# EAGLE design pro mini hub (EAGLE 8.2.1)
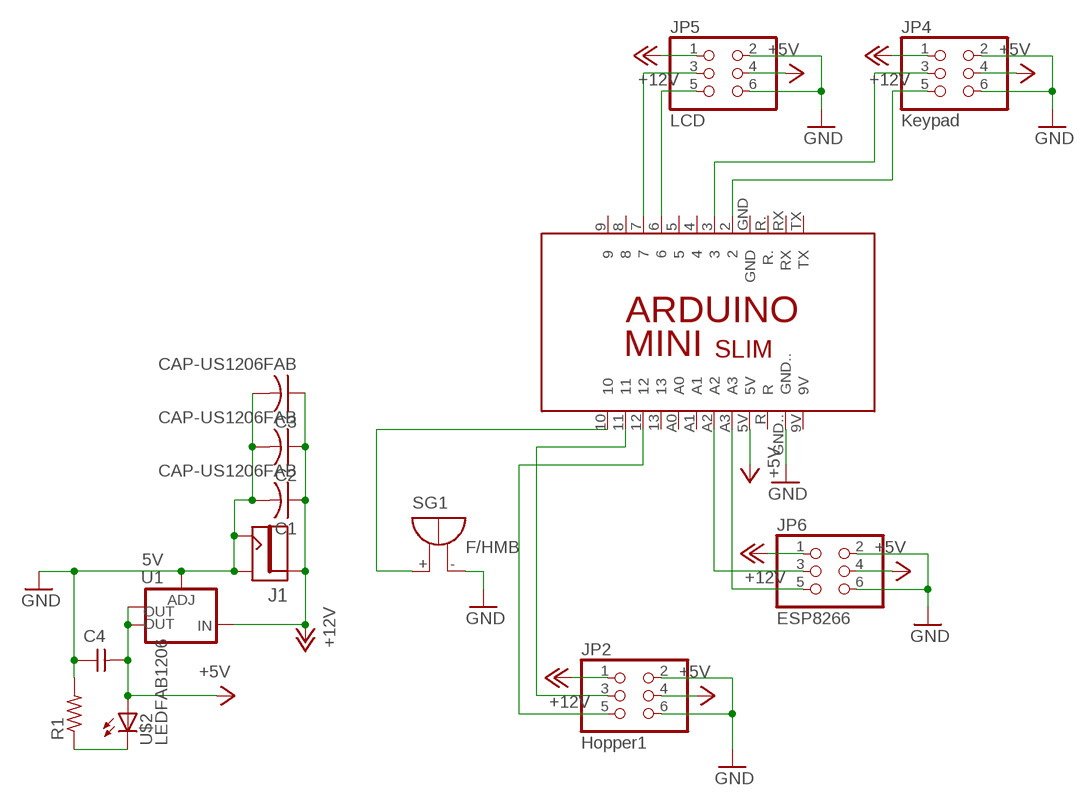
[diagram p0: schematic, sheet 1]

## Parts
C1  CAP-US1206FAB  [C1206FAB]
C2  CAP-US1206FAB  [C1206FAB]
C3  CAP-US1206FAB  [C1206FAB]
C4  CAP-UNPOLARIZEDFAB  [C1206FAB]
J1  JACK2.1MM  [JACK_2.1MM]
JP2  Hopper1  PINHD-2X3-SMD  [2X03SMD]
JP4  Keypad  PINHD-2X3-SMD  [2X03SMD]
JP5  LCD  PINHD-2X3-SMD  [2X03SMD]
JP6  ESP8266  PINHD-2X3-SMD  [2X03SMD]
PCB1  ARDUINO_MINI_SLIM  [ARDUINO_MINI_SLIM]
R1  RES-US1206FAB  [R1206FAB]
SG1  F/HMB  [F/HMB]
U1  5V  V_REG_LM1117SOT223  [SOT223]
U$2  LEDFAB1206  [LED1206FAB]

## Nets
+5V: C4.2 JP2.4 JP4.4 JP5.4 JP6.4 PCB1.5V U1.2(OUT) U1.4(OUT) U$2.1(A)
+12V: C1.1 C2.1 C3.1 J1.PIN JP2.1 JP4.1 JP5.1 JP6.1 U1.3(IN)
GND: C1.2 C2.2 C3.2 C4.1 J1.CONTACT J1.SHUNT JP2.2 JP2.6 JP4.2 JP4.6 JP5.2 JP5.6 JP6.2 JP6.6 PCB1.GND.. R1.2 SG1.- U1.1(ADJ)
N$1: PCB1.10 SG1.+
N$2: R1.1 U$2.2(C)
N$3: JP2.3 PCB1.11
N$4: JP2.5 PCB1.12
N$5: JP6.5 PCB1.A3
N$6: JP6.3 PCB1.A2
N$7: JP5.5 PCB1.6
N$8: JP5.3 PCB1.7
N$9: JP4.5 PCB1.2
N$10: JP4.3 PCB1.3
Unconnected: PCB1.4 PCB1.5 PCB1.8 PCB1.9 PCB1.9V PCB1.13 PCB1.A0 PCB1.A1 PCB1.GND PCB1.R PCB1.R. PCB1.RX PCB1.TX

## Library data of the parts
C1-C3 = fab:CAP-US
C4 = fab:CAP-UNPOLARIZED
J1 = fab:JACK
JP2 JP4-JP6 = fab:PINHD-2X3-SMD: PIN HEADER
PCB1 = E14_Arduino_revC:ARDUINO_MINI_SLIM: Device for representing an Arduino Mini board with a footprint in an EAGLE design. Created by Dave Young for Element14. More EAGLE documentation at: http://www.element14.com/community/community/knode/cadsoft_eagle
R1 = fab:RES-US: Resistor (US Symbol)
SG1 = buzzer:F/HMB: BUZZER; OC_FARNELL: unknown; OC_NEWARK: unknown
U1 = fab:V_REG_LM1117: Voltage Regulator LM1117 Standard adjustable voltage regulator but in SMD form. Spark Fun Electronics SKU : COM-00595; PROD_ID: VREG-08170
U$2 = fab:LED: LED

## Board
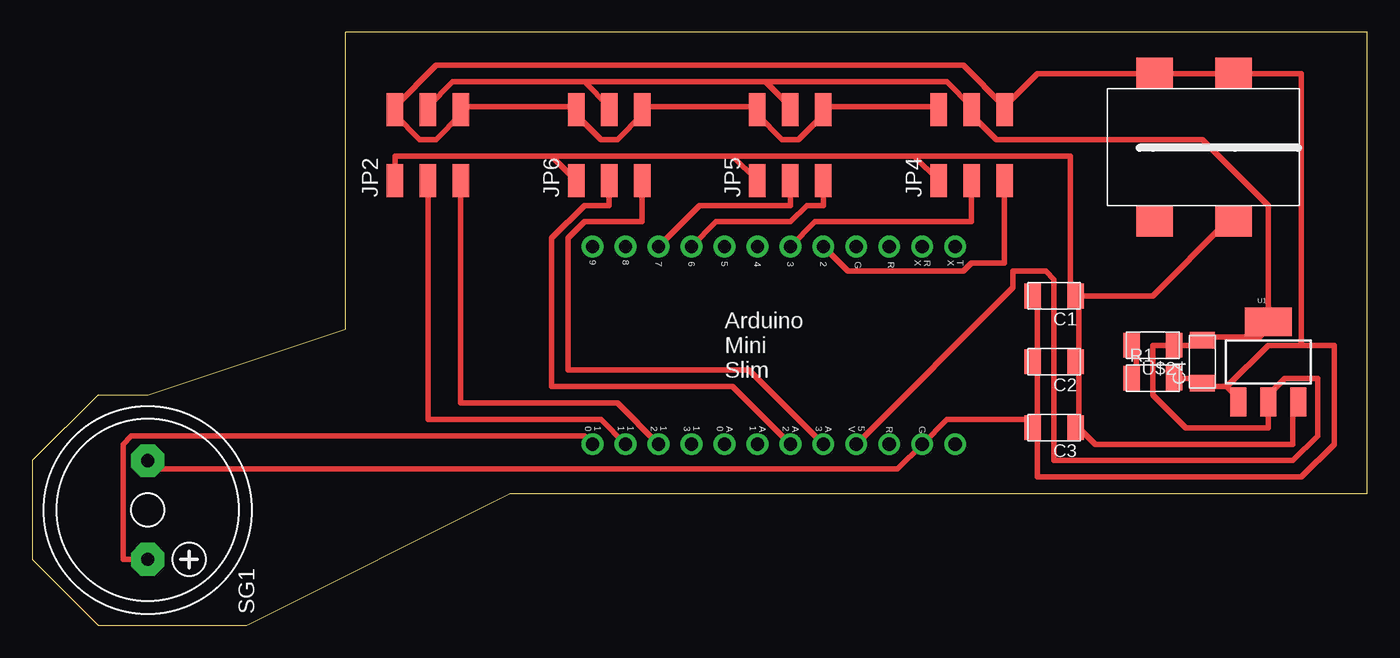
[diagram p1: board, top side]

Size 102.87 x 45.72 mm. Coordinates in mm from the lower left corner, seen from the top.
Outline: 5.08,17.78 0,12.7 0,5.08 5.08,0 16.51,0 36.83,10.16 102.87,10.16 102.87,45.72 24.13,45.72 24.13,22.86 8.89,17.78 5.08,17.78
Copper layers (1*16): Top 0.035mm / dielectric 1.5mm / Bottom 0.035mm
Design rules "default *": minimum track width 16mil, minimum drill 0.35mm, track to track 16mil, track to pad 16mil, pad to pad 16mil, via to via 16mil, smd to smd 16mil, copper to edge 40mil, drill to drill 6mil, minimum pad ring 10mil, minimum via ring 8mil, stop-mask expansion 4mil, vias tented up to drill 0mil, thermal gap 10mil

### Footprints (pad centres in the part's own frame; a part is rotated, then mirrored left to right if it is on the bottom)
C1206FAB = smd 1.27 x 1.905: 1 -1.651,0; 2 1.651,0
JACK_2.1MM = smd 2.388 x 2.794: CONTACT 5.766,-2.413; PIN -5.639,-2.413; PIN1 -5.639,3.683; SHUNT 5.766,3.683
2X03SMD = smd 2.54 x 1.27: 1 -2.54,2.54; 2 2.92,2.54; 3 -2.54,0; 4 2.92,0; 5 -2.54,-2.54; 6 2.92,-2.54
ARDUINO_MINI_SLIM = drill 1.016 pad 1.676: 2 19.05,16.51; 3 16.51,16.51; 4 13.97,16.51; 5 11.43,16.51; 5V 21.59,1.27; 6 8.89,16.51; 7 6.35,16.51; 8 3.81,16.51; 9 1.27,16.51; 9V 29.21,1.27; 10 1.27,1.27; 11 3.81,1.27; 12 6.35,1.27; 13 8.89,1.27; A0 11.43,1.27; A1 13.97,1.27; A2 16.51,1.27; A3 19.05,1.27; GND 21.59,16.51; GND.. 26.67,1.27; R 24.13,1.27; R. 24.13,16.51; RX 26.67,16.51; TX 29.21,16.51
R1206FAB = smd 1.27 x 1.905: 1 -1.651,0; 2 1.651,0
F/HMB = drill 1.016 pad 2.54 octagon: + 3.81,0; - -3.81,0
SOT223 = smd 1.219 x 2.235: 1 -2.311,-3.099; 2 0,-3.099; 3 2.311,-3.099 | smd 3.6 x 2.2: 4 0,3.099
LED1206FAB = smd 1.27 x 1.905: 1 -1.651,0; 2 1.651,0

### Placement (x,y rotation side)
C1  78.74,25.4 180 top
C2  78.74,20.32 180 top
C3  78.74,15.24 180 top
C4  90.17,20.32 90 top
J1  90.17,36.83 90 top
JP2  30.48,36.83 90 top
JP4  72.39,36.83 90 top
JP5  58.42,36.83 90 top
JP6  44.45,36.83 90 top
PCB1  41.91,12.7 0 top
R1  86.36,19.05 0 top
SG1  8.89,8.89 270 top
U1  95.25,20.32 0 top
U$2  86.36,21.59 180 top

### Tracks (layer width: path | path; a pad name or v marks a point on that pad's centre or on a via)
+5V
  Top 0.406: 42.55,41.91 32.38,41.91 30.48,40.01 JP2.4 | 42.55,41.91 44.45,40.01 JP6.4 | 56.52,41.91 58.42,40.01 JP5.4 | 42.55,41.91 56.52,41.91 | 56.52,41.91 70.48,41.91 72.39,40.01 JP4.4 72.39,39.37 74.3,37.47 90.17,37.47 95.25,32.38 U1.4 95.25,22.86 94.62,22.23 90.17,22.23 C4.2 90.17,21.59 U$2.1 86.36,21.59 86.36,17.78 88.9,15.24 95.25,15.24 U1.2 95.25,17.78 96.52,19.05 99.06,19.05 99.06,14.61 97.16,12.7 78.74,12.7 78.74,26.67 78.11,27.3 75.57,27.3 75.57,26.04 PCB1.5V
+12V
  Top 0.406: 80.65,20.32 80.65,15.24 | 80.65,20.32 80.65,25.4 | 80.65,20.32 C2.1 | 80.65,15.24 81.92,13.97 97.16,13.97 97.16,17.14 U1.3 | 80.65,15.24 C3.1 | 80.65,25.4 86.36,25.4 92.08,31.12 J1.PIN | 80.65,25.4 C1.1 80.01,25.4 80.01,36.2 67.95,36.2 | JP2.1 27.94,36.2 40,36.2 | JP6.1 40,36.2 | 53.98,36.2 JP5.1 | 40,36.2 53.98,36.2 | 67.95,36.2 JP4.1 | 53.98,36.2 67.95,36.2
GND
  Top 0.406: 77.47,20.32 77.47,15.88 | 77.47,15.88 77.47,15.24 | 77.47,20.32 77.47,25.4 C1.2 | 77.47,20.32 C2.2 | 77.47,15.88 70.48,15.88 PCB1.GND.. 66.68,12.07 9.53,12.07 SG1.- | 77.47,15.88 C3.2 77.47,15.24 | JP4.2 69.85,40.01 60.96,40.01 JP5.6 60.96,39.37 59.05,37.47 57.79,37.47 55.88,39.37 JP5.2 55.88,40.01 46.99,40.01 JP6.6 46.99,39.37 45.09,37.47 43.81,37.47 41.91,39.37 JP6.2 41.91,40.01 33.02,40.01 JP2.6 33.02,39.37 31.12,37.47 29.84,37.47 27.94,39.37 JP2.2 27.94,40.01 31.12,43.18 71.76,43.18 74.93,40.01 | R1.2 90.17,19.05 C4.1 90.17,18.41 92.08,18.41 | 92.08,18.41 92.71,17.78 U1.1 | 74.93,40.01 77.47,42.55 86.36,42.55 J1.SHUNT 87,42.55 92.08,42.55 J1.CONTACT 92.71,42.55 97.79,42.55 97.79,21.59 | 92.08,18.41 95.25,21.59 97.79,21.59 | 74.93,40.01 JP4.6 | 77.47,15.24 77.47,11.43 97.79,11.43 100.33,13.97 100.33,21.59 97.79,21.59
N$1
  Top 0.406: PCB1.10 42.55,14.61 7.62,14.61 6.99,13.97 6.99,5.08 SG1.+
N$2
  Top 0.406: R1.1 85.09,19.05 85.09,21.59 U$2.2
N$3
  Top 0.406: JP2.3 30.48,15.88 43.81,15.88 PCB1.11
N$4
  Top 0.406: JP2.5 33.02,17.14 45.09,17.14 PCB1.12
N$5
  Top 0.406: JP6.5 46.99,31.12 42.55,31.12 41.27,29.84 41.27,19.68 55.24,19.68 PCB1.A3
N$6
  Top 0.406: JP6.3 44.45,32.38 42.55,32.38 40,29.84 40,18.41 53.98,18.41 PCB1.A2
N$7
  Top 0.406: JP5.5 60.96,32.38 59.69,32.38 58.42,31.12 52.7,31.12 PCB1.6
N$8
  Top 0.406: JP5.3 58.42,32.38 51.43,32.38 PCB1.7
N$9
  Top 0.406: JP4.5 74.93,27.94 72.39,27.94 71.76,27.3 62.87,27.3 PCB1.2
N$10
  Top 0.406: JP4.3 72.39,31.12 60.32,31.12 PCB1.3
